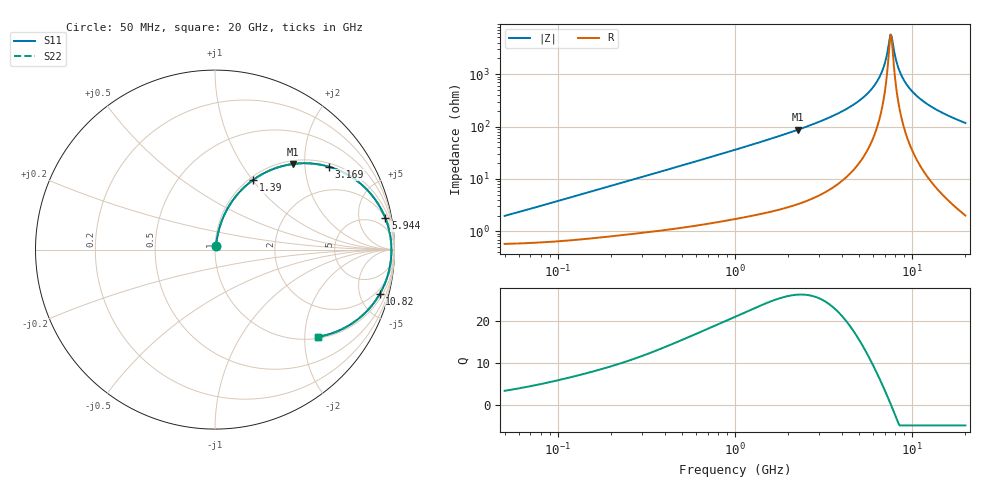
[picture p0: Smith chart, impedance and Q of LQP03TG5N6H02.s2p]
!Murata Part Number: LQP03TG5N6H02
!These Parameters are Measured in Series Mode Connection
!  o--[Z]--o
!Port1  Port2
!  o-------o
!Freq. Start=50[MHz] Stop=20[GHz], 401[Steps]
# Hz S RI R 50
!Freq.(Hz) S11(Real) S11(Imag) S21(Real) S21(Imag) S12(Real) S12(Imag) S22(Real) S22(Imag)
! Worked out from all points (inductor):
!   401 points, 50 MHz to 20 GHz, reference 50 ohm
!   read as one part in series: L = 6 nH near 51.52 MHz
!   highest Q = 26.3 at 2.279 GHz (marker M1), where L = 6.11 nH
!   self-resonance near 7.554 GHz
!   S11 on the Smith chart (normalised r, x): 50 MHz: 1.01, +0.04; 1.39 GHz: 1.04, +1.01; 3.169 GHz: 1.11, +2.67; 5.944 GHz: 2, +11; 10.82 GHz: 1.41, -7.26; 20 GHz: 1.04, -2.34
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5e7  0.00608 0.0187  0.9939 -0.0187  0.9939 -0.0187  0.00608 0.0187
1.364002e8  0.00952 0.0499  0.9905 -0.0499  0.9905 -0.0499  0.00952 0.0499
3.721004e8  0.0275 0.1298  0.9725 -0.1298  0.9725 -0.1298  0.0275 0.1298
1e9  0.1262 0.3091  0.8738 -0.3091  0.8738 -0.3091  0.1262 0.3091
1.390315e9  0.2136 0.3893  0.7864 -0.3893  0.7864 -0.3893  0.2136 0.3893
2.279204e9  0.4363 0.4773  0.5637 -0.4773  0.5637 -0.4773  0.4363 0.4773
2.728004e9  0.5428 0.4793  0.4572 -0.4793  0.4572 -0.4793  0.5428 0.4793
3.168813e9  0.6363 0.4614  0.3637 -0.4614  0.3637 -0.4614  0.6363 0.4614
4.608136e9  0.8523 0.328  0.1477 -0.328  0.1477 -0.328  0.8523 0.328
5.944466e9  0.9495 0.174  0.0505 -0.174  0.0505 -0.174  0.9495 0.174
6.406762e9  0.9666 0.1222  0.0334 -0.1222  0.0334 -0.1222  0.9666 0.1222
6.802353e9  0.976 0.0795  0.024 -0.0795  0.024 -0.0795  0.976 0.0795
7.114996e9  0.9805 0.047  0.0195 -0.047  0.0195 -0.047  0.9805 0.047
7.442007e9  0.9828 0.0142  0.0172 -0.0142  0.0172 -0.0142  0.9828 0.0142
7.668323e9  0.9831 -0.00773  0.0169 0.00773  0.0169 0.00773  0.9831 -0.00773
7.784049e9  0.9829 -0.0187  0.0171 0.0187  0.0171 0.0187  0.9829 -0.0187
8.264682e9  0.9796 -0.0625  0.0204 0.0625  0.0204 0.0625  0.9796 -0.0625
8.907419e9  0.9699 -0.1164  0.0301 0.1164  0.0301 0.1164  0.9699 -0.1164
9.745021e9  0.9504 -0.1792  0.0496 0.1792  0.0496 0.1792  0.9504 -0.1792
1.082228e10  0.9174 -0.2482  0.0826 0.2482  0.0826 0.2482  0.9174 -0.2482
1.417136e10  0.7898 -0.3928  0.2102 0.3928  0.2102 0.3928  0.7898 -0.3928
2e10  0.5762 -0.4856  0.4238 0.4856  0.4238 0.4856  0.5762 -0.4856
